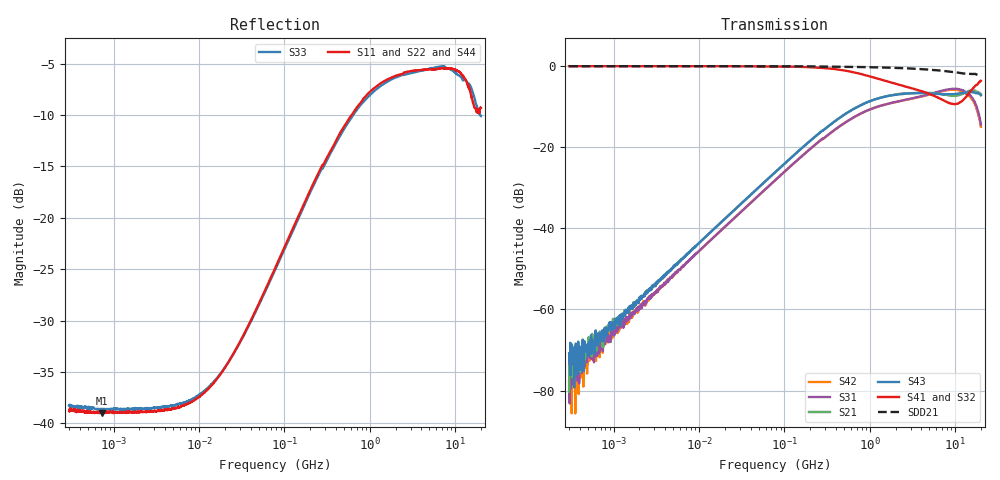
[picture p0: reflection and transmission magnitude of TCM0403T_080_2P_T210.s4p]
! S-Parameter Data Generated by TDK Corporation
! Copyright(C) 2024 TDK Corporation.
! All Rights Reserved.
! TDK P/N: TCM0403T-080-2P-T210 (Signal Line Common Mode Choke/Filter)
! Property: -
! Size(LxWxT): 0.45x0.3x0.23mm
! Model Type: s2p (Touchstone File Format Version 1.0)
! Frequency: DC=Yes Start=0.3MHz Stop=20000MHz 1602points Log-sweep
! Model Generated on May 28, 2024
! Terms and conditions regarding TDK Simulation Models:
! 1)This simulation model is being provided solely for informational
!  purposes. Please refer to the specifications of the products in
!  terms of detailed characteristics of such products.
! 2)In no event shall TDK Corporation of any of its subsidiaries be
!  liable for any loss or damage arising, directly or indirectly,
!  from any information contained in this simulation model, including,
!  but not limited to loss or damages arising from any inaccuracies,
!  omissions or errors in connection with such information.
! 3)Any and all copyrights on this simulation model are owned by
!  TDK Corporation.  Duplication or redistribution of this simulation
!  model without prior written permission from TDK Corporation
!  is prohibited.
! 4)This simulation model is subject to any modification or change
!  without any prior notice.
! 5)Neither TDK Corporation nor any of its subsidiaries shall make any
!  warranty, express or implied, including but not limited to the
!  correctness, implied warranties of merchantability and fitness for
!  a particular purpose with respect to this simulation models.
! 6)The use of this simulation model shall be deemed to have consented
!  to the terms and conditions hereof.
! Port Assignments:
!  1 ---@@@--- 4
!  2 ---@@@--- 3
! Applicable Conditions:
!  Temperature = 25 degC
!  DC Bias Current = 0 A
!  Small Signal Operation
# Hz S MA R 50
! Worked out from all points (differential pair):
!   1601 points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, 300 kHz to 20 GHz, reference 50 ohm
!   strongest paths, dB at 300 kHz, 4.882 MHz, 77.46 MHz, 1.261 GHz, 20 GHz:
!     S41: -0.1, -0.1, -0.1, -3.2, -3.7
!     S32: -0.1, -0.1, -0.2, -3.1, -3.6
!     S43: -70.8, -49.9, -26.2, -8.0, -7.3
!     S21: -80.3, -49.9, -26.2, -8.0, -7.0
!     S31: -77.8, -51.8, -28.2, -10.0, -14.5
!     S42: -74.1, -52.1, -28.2, -10.0, -15.0
!   taken as a pair (ports 1,2 in; 4,3 out), SDD21 dB: -0.1, -0.1, -0.1, -0.4, -2.4
!   lowest |S11| = -39.0 dB at 726.9 kHz (marker M1), VSWR 1.02, Z = 51.1 - j0.00191 ohm
!   |S11| at or under -10 dB: start of sweep to 613.2 MHz
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300000  0.01146 -3.6  0.0001151 51.5  0.000205 -104.7  0.9883 0.0
        9.633e-05 44.6  0.01189 1.2  0.988 -0.0  0.0001715 -112.0
        0.0001289 -129.9  0.9879 -0.0  0.01222 0.4  0.0001793 80.9
        0.9891 -0.0  0.000197 -116.5  0.0002889 66.8  0.0111 0.1
726922  0.0112 -0.1  0.0005348 92.3  0.0004357 -101.6  0.9887 -0.0
        0.000459 92.1  0.01173 2.3  0.9882 -0.0  0.0003746 -82.6
        0.0003509 -87.1  0.9882 -0.0  0.01184 2.1  0.0004819 83.2
        0.9889 -0.1  0.0003342 -82.3  0.0004415 95.5  0.01121 2.3
1.442434e7  0.01557 41.9  0.009462 87.7  0.007529 -92.7  0.9883 -0.7
            0.009449 87.8  0.0157 40.0  0.988 -0.7  0.007535 -92.7
            0.007532 -92.6  0.988 -0.7  0.01574 40.2  0.009462 87.7
            0.9884 -0.7  0.007525 -92.6  0.009456 87.6  0.01553 42.1
6.247594e8  0.3196 47.5  0.2887 50.0  0.2266 -141.3  0.8374 -22.7
            0.2888 50.0  0.3118 48.1  0.8424 -21.9  0.2266 -141.0
            0.227 -141.3  0.8424 -21.9  0.3122 47.8  0.2881 49.8
            0.8387 -22.7  0.2269 -140.7  0.2881 49.8  0.323 47.8
3.078648e9  0.5167 6.4  0.4608 8.3  0.3965 139.2  0.5284 -51.2
            0.4609 8.3  0.5079 7.5  0.5395 -50.9  0.3922 140.4
            0.3957 139.4  0.5387 -50.9  0.5063 5.5  0.4592 8.9
            0.5293 -51.0  0.3932 140.4  0.4591 8.9  0.5227 6.7
1.048674e10  0.5222 -29.0  0.4303 -11.2  0.5228 28.1  0.3382 -177.4
             0.4305 -11.3  0.5439 -31.0  0.3362 -179.4  0.5038 29.5
             0.5186 28.1  0.3341 -179.4  0.5004 -35.2  0.4534 -9.9
             0.3403 -176.4  0.5067 30.0  0.4529 -9.8  0.5292 -30.8
2e10  0.3418 -51.0  0.4458 -45.3  0.1908 -67.1  0.6461 54.4
      0.4454 -45.5  0.3104 -54.7  0.6672 52.0  0.1749 -60.6
      0.1881 -66.4  0.6625 52.6  0.3123 -71.6  0.4316 -37.8
      0.6532 53.6  0.1786 -64.5  0.4323 -37.4  0.4203 -66.4
